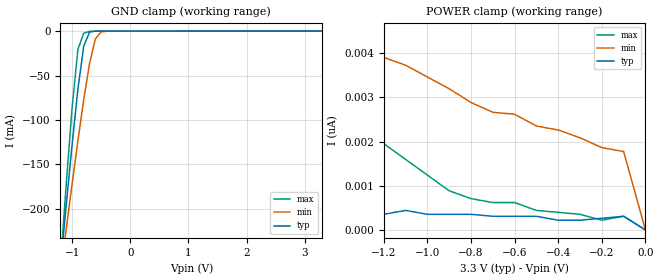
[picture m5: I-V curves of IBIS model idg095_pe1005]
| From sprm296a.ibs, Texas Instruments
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[Model]   idg095_pe1005
Model_type   Input
| Input with 100 UA PULLDOWN
Polarity   Non-Inverting
| signals   A, Y
Vinl = 0.8V
Vinh = 2.0V
|   typ   min   max
C_comp   3.069p   3.031p   3.089p
|   typ   min   max
[Temperature Range]   25   -40   125
|   typ   min   max
[Voltage Range]   3.30V   3.00V   3.60V
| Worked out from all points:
|   GND clamp passes 1 mA (typ) near -0.69 V on its own axis
[GND_clamp]
|   Voltage   I(typ)   I(min)   I(max)
-3.3V     -1.821A    -1.4A      -2.329A
-1.2V     -265.5mA   -273.8mA   -263.6mA
-1.1V     -195.6mA   -222.6mA   -172.1mA
-1V       -128.2mA   -172.4mA   -86.53mA
-900mV    -65.62mA   -123.6mA   -20.66mA
-800mV    -17.04mA   -77.38mA   -2.347mA
-700mV    -1.069mA   -36.57mA   -290.5uA
-600mV    -73.43uA   -8.795mA   -63.99uA
-500mV    -27uA      -787.1uA   -42.16uA
-300mV    -14.39uA   -10.5uA    -24.27uA
3.3V      37.64uA    18.83uA    71.45uA
[POWER_clamp]
|   Voltage   I(typ)   I(min)   I(max)
-3.3V     6.306nA    22.2nA     577.9nA
-3.1V     4.885nA    18.56nA    335.7nA
-2.7V     2.931nA    13.5nA     112.4nA
-2.6V     2.309nA    12.26nA    85.18nA
-2.2V     1.243nA    8.882nA    28.24nA
-1.6V     710.5pA    5.418nA    5.418nA
-1.5V     621.7pA    5.063nA    4.174nA
-1.4V     621.7pA    4.707nA    3.197nA
-1.2V     355.3pA    3.908nA    1.954nA
-900mV    355.3pA    3.197nA    888.2pA
-100mV    310.9pA    1.776nA    310.9pA
0V        1pA        1pA        1pA
